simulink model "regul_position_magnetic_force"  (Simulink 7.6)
settings: Solver=ode15s  StartTime=0.0  StopTime=50  RelTol=1e-3
StopFcn:
  | close all
  | load signaux_regul.mat
  | plot(xyz(1,:),xyz(3,:))
  | hold on
  | plot(xyz(1,:),xyz(4,:))
  | axis([5 50 0 2])
  | xlabel('temps')
  | grid
  | title('Consigne et position de la masse')
  | figure
  | plot(xyz(1,:),xyz(2,:))
  | grid
  | title('Signal de commande')
  | axis([5 50 -0.015 0.015])
  | xlabel('temps')
undefined symbols (not defined in the file or in its folder): sigbuilder_block
libraries: fl_lib x17, nesl_utility x6

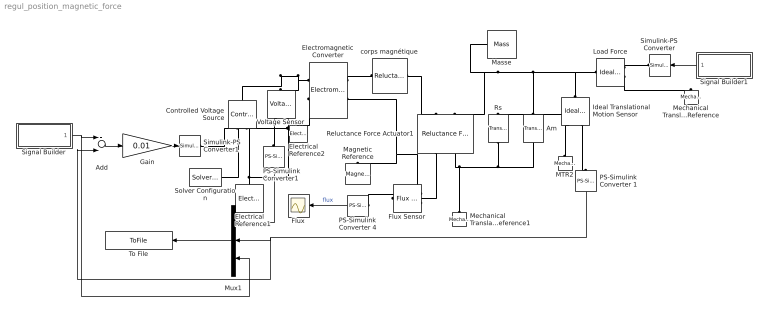
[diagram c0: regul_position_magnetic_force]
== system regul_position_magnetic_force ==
  Add : Sum  Inputs=+-
  Am : fl_lib/Mechanical/Translational Elements/Translational Damper  DialogController=NetworkEngine.DynNeDlgSource  SystemSampleTime=-1  D=10 N/(m/s)  f_Log=off  v_Log=off  LocalVarNames=|force|rel_velocity|power  LocalVarDescs=|Damping force (N)|Damper relative velocity (m/s)|Power dissipated in the damper (W)  LocalVarLogging=[0 0 0]
  Controlled Voltage Source : fl_lib/Electrical/Electrical Sources/Controlled Voltage Source  DialogController=NetworkEngine.DynNeDlgSource  SystemSampleTime=-1  i_Log=off  v_Log=off  LocalVarNames=|i|v  LocalVarDescs=|i|v  LocalVarLogging=[0 0]
  Electrical  Reference1 : fl_lib/Electrical/Electrical Elements/Electrical Reference  DialogController=NetworkEngine.DynNeDlgSource  SystemSampleTime=-1  i_Log=off  LocalVarNames=|i  LocalVarDescs=|i  LocalVarLogging=0
  Electrical Reference2 : fl_lib/Electrical/Electrical Elements/Electrical Reference  DialogController=NetworkEngine.DynNeDlgSource  SystemSampleTime=-1  i_Log=off  LocalVarNames=|i  LocalVarDescs=|i  LocalVarLogging=[]
  Electromagnetic Converter : fl_lib/Magnetic/Magnetic Elements/Electromagnetic Converter  DialogController=NetworkEngine.DynNeDlgSource  SystemSampleTime=-1  Nw=2000  i_Log=off  v_Log=off  mmf_Log=off  phi_Log=off  LocalVarNames=|i|v|mmf|phi  LocalVarDescs=|i|v|mmf|phi  LocalVarLogging=[0 0 0 0]
  Flux : Scope
  Flux Sensor : fl_lib/Magnetic/Magnetic Sensors/Flux Sensor  DialogController=NetworkEngine.DynNeDlgSource  SystemSampleTime=-1  phi_Log=off  mmf_Log=off  LocalVarNames=|phi|mmf  LocalVarDescs=|phi|mmf  LocalVarLogging=[0 0]
  Gain : Gain  Gain=0.01
  Ideal Translational Motion Sensor : fl_lib/Mechanical/Mechanical Sensors/Ideal Translational Motion Sensor  DialogController=NetworkEngine.DynNeDlgSource  SystemSampleTime=-1  offset=5 mm  v_Log=off  f_Log=off  x_Log=off  LocalVarNames=|v|f|x  LocalVarDescs=|v|f|x  LocalVarLogging=[]
  Load Force : fl_lib/Mechanical/Mechanical Sources/Ideal Force Source  DialogController=NetworkEngine.DynNeDlgSource  SystemSampleTime=-1  v_Log=off  f_Log=off  LocalVarNames=|force|rel_velocity|power  LocalVarDescs=|Force (N)|Relative velocity (m/s)|Power generated by the source (W)  LocalVarLogging=[0 0 0]
  MTR2 : fl_lib/Mechanical/Translational Elements/Mechanical Translational Reference  Tag=Factory Generic  DialogController=NetworkEngine.DynNeDlgSource  SystemSampleTime=-1  f_Log=off  LocalVarNames=|f  LocalVarDescs=|f  LocalVarLogging=[]
  Magnetic Reference : fl_lib/Magnetic/Magnetic Elements/Magnetic Reference  DialogController=NetworkEngine.DynNeDlgSource  SystemSampleTime=-1  phi_Log=off  LocalVarNames=|phi  LocalVarDescs=|phi  LocalVarLogging=0
  Masse : fl_lib/Mechanical/Translational Elements/Mass  DialogController=NetworkEngine.DynNeDlgSource  SystemSampleTime=-1  mass=1 kg  initial_velocity=0 m/s  f_Log=off  LocalVarNames=|force|velocity  LocalVarDescs=|Inertia force (N)|Mass absolute velocity (m/s)  LocalVarLogging=[0 0]
  Mechanical Translational Reference : fl_lib/Mechanical/Translational Elements/Mechanical Translational Reference  DialogController=NetworkEngine.DynNeDlgSource  SystemSampleTime=-1  f_Log=off  LocalVarNames=|f  LocalVarDescs=|f  LocalVarLogging=[]
  Mechanical Translational Reference1 : fl_lib/Mechanical/Translational Elements/Mechanical Translational Reference  DialogController=NetworkEngine.DynNeDlgSource  SystemSampleTime=-1  f_Log=off  LocalVarNames=|f  LocalVarDescs=|f  LocalVarLogging=[]
  Mux1 : Mux  Inputs=3
  PS-Simulink Converter 1 : nesl_utility/PS-Simulink Converter  DialogController=NetworkEngine.DynNeUtilDlgSource  SystemSampleTime=-1  PhysicalDomain=network_engine_domain  LeftPortType=input  RightPortType=output  SubClassName=ps_output  Unit=mm  AffineConversion=off
  PS-Simulink Converter 4 : nesl_utility/PS-Simulink Converter  DialogController=NetworkEngine.DynNeUtilDlgSource  SystemSampleTime=-1  PhysicalDomain=network_engine_domain  LeftPortType=input  RightPortType=output  SubClassName=ps_output  Unit=Wb  AffineConversion=off
  PS-Simulink Converter1 : nesl_utility/PS-Simulink Converter  DialogController=NetworkEngine.DynNeUtilDlgSource  SystemSampleTime=-1  PhysicalDomain=network_engine_domain  LeftPortType=input  RightPortType=output  SubClassName=ps_output  Unit=1  AffineConversion=off
  Reluctance Force Actuator1 : fl_lib/Magnetic/Magnetic Elements/Reluctance Force Actuator  DialogController=NetworkEngine.DynNeDlgSource  SystemSampleTime=-1  x0=5 mm  xmin=1e-9 mm  CSA=4 cm^2  mur=1  K_contact=1e6 N/m  D_contact=50 N/(m/s)  mmf_Log=off  phi_Log=off  f_Log=off  u_Log=off  x_Log=off  LocalVarNames=|mmf|phi|f|u|x  LocalVarDescs=|mmf|phi|f|u|x  LocalVarLogging=[0 0 0 0 0]
  Rs : fl_lib/Mechanical/Translational Elements/Translational Spring  DialogController=NetworkEngine.DynNeDlgSource  SystemSampleTime=-1  spr_rate=150 N/m  init_def=0 mm  f_Log=off  v_Log=off  x_Log=off  LocalVarNames=|force|deformation  LocalVarDescs=|Spring force (N)|Spring deformation (m)  LocalVarLogging=[0 0]
  Signal Builder : Subsystem  Tag=STV Subsys  LoadFcn=sigbuilder_block('load');  StartFcn=sigbuilder_block('start');  StopFcn=sigbuilder_block('stop');  ClipboardFcn=sigbuilder_block('clipboard');
  Signal Builder1 : Subsystem  Tag=STV Subsys  LoadFcn=sigbuilder_block('load');  StartFcn=sigbuilder_block('start');  StopFcn=sigbuilder_block('stop');  ClipboardFcn=sigbuilder_block('clipboard');
  Simulink-PS Converter : nesl_utility/Simulink-PS Converter  DialogController=NetworkEngine.DynNeUtilDlgSource  SystemSampleTime=-1  PhysicalDomain=network_engine_domain  LeftPortType=input  RightPortType=output  SubClassName=ps_input  Unit=1  AffineConversion=off  InputFilterTimeConstant=.001  UdotUserProvided=0
  Simulink-PS Converter1 : nesl_utility/Simulink-PS Converter  DialogController=NetworkEngine.DynNeUtilDlgSource  SystemSampleTime=-1  PhysicalDomain=network_engine_domain  LeftPortType=input  RightPortType=output  SubClassName=ps_input  Unit=1  AffineConversion=off  InputFilterTimeConstant=.001  UdotUserProvided=0
  Solver Configuration : nesl_utility/Solver Configuration  DialogController=NetworkEngine.DynNeUtilDlgSource  SystemSampleTime=-1  PhysicalDomain=network_engine_domain  LeftPortType=input  RightPortType=generic  SubClassName=solver  Accelerate=off  Profile=off  ResidualTolerance=1e-9  MaxNonlinIter=3  MaxModeIter=2  DoFixedCost=off  UseLocalSampling=off  DoDC=off  LinearAlgebra=Sparse  LocalSolverSampleTime=.001  LocalSolverChoice=NE_BACKWARD_EULER_ADVANCER  UseLocalSolver=off
  To File : ToFile  Filename=signaux_regul.mat  MatrixName=xyz
  Voltage Sensor : fl_lib/Electrical/Electrical Sensors/Voltage Sensor  DialogController=NetworkEngine.DynNeDlgSource  SystemSampleTime=-1  i1_Log=off  v1_Log=off  LocalVarNames=|i1|v1  LocalVarDescs=|i1|v1  LocalVarLogging=[0 0]
  corps magnétique : fl_lib/Magnetic/Magnetic Elements/Reluctance  DialogController=NetworkEngine.DynNeDlgSource  SystemSampleTime=-1  g=10 cm  CSA=10 cm^2  mur=50000  phi_Log=off  mmf_Log=off  LocalVarNames=|phi|mmf  LocalVarDescs=|phi|mmf  LocalVarLogging=[0 0]
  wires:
  PS-Simulink Converter 4/1 -> Flux/1  "flux"
  Signal Builder1/1(Signal 1) -> Simulink-PS Converter/1
  PS-Simulink Converter1/1 -> Mux1/1
  PS-Simulink Converter 1/1 -> Mux1/2, Add/2
  Add/1 -> Gain/1
  Signal Builder/1(Signal 1) -> Add/1, Mux1/3
  Gain/1 -> Simulink-PS Converter1/1
  Mux1/1 -> To File/1
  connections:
  PS-Simulink Converter 4/LConn1 -- Flux Sensor/RConn1
  Load Force/RConn2 -- Mechanical Translational Reference/LConn1
  Ideal Translational Motion Sensor/RConn3 -- PS-Simulink Converter 1/LConn1
  Electromagnetic Converter/RConn1 -- corps magnétique/LConn1
  corps magnétique/RConn1 -- Reluctance Force Actuator1/LConn1
  Flux Sensor/RConn2 -- Electromagnetic Converter/RConn2 -- Magnetic Reference/LConn1
  Masse/LConn1 -- Reluctance Force Actuator1/LConn2 -- Rs/LConn1 -- Am/LConn1 -- Load Force/LConn1 -- Ideal Translational Motion Sensor/LConn1
  Load Force/RConn1 -- Simulink-PS Converter/RConn1
  Electromagnetic Converter/LConn1 -- Voltage Sensor/LConn1 -- Controlled Voltage Source/LConn1
  Voltage Sensor/RConn2 -- Solver Configuration/RConn1 -- Controlled Voltage Source/RConn2 -- Electrical  Reference1/LConn1
  PS-Simulink Converter1/LConn1 -- Voltage Sensor/RConn1
  MTR2/LConn1 -- Ideal Translational Motion Sensor/RConn1
  Simulink-PS Converter1/RConn1 -- Controlled Voltage Source/RConn1
  Electromagnetic Converter/LConn2 -- Electrical Reference2/LConn1
  Rs/RConn1 -- Mechanical Translational Reference1/LConn1 -- Reluctance Force Actuator1/RConn2 -- Am/RConn1
  Reluctance Force Actuator1/RConn1 -- Flux Sensor/LConn1

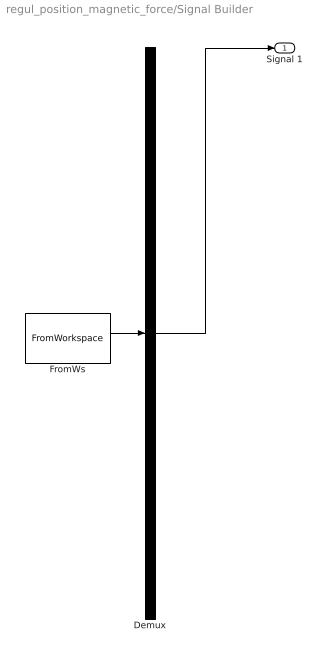
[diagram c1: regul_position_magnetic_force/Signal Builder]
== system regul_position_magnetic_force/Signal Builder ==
  Demux : Demux  Tag=STV Demux  Outputs=1
  FromWs : FromWorkspace  Tag=STV FromWs  VariableName=tuvar  SampleTime=0  SigBuilderData=DataTag0  VnvData=DataTag1
  Signal 1 : Outport  Tag=STV Outport
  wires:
  Demux/1 -> Signal 1/1
  FromWs/1 -> Demux/1

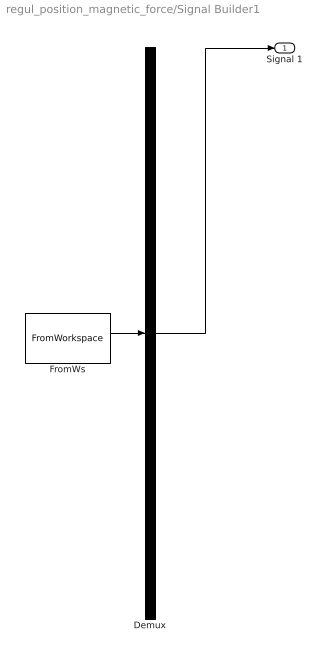
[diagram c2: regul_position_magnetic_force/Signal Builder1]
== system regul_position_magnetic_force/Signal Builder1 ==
  Demux : Demux  Tag=STV Demux  Outputs=1
  FromWs : FromWorkspace  Tag=STV FromWs  VariableName=tuvar  SampleTime=0  SigBuilderData=DataTag2  VnvData=DataTag3
  Signal 1 : Outport  Tag=STV Outport
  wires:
  FromWs/1 -> Demux/1
  Demux/1 -> Signal 1/1
